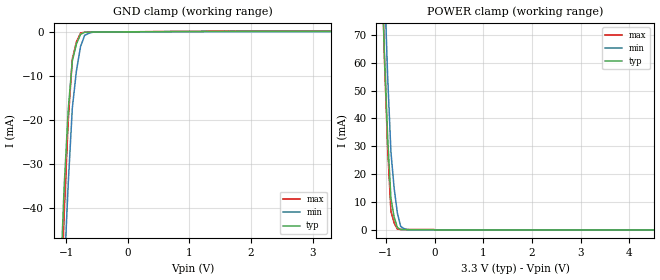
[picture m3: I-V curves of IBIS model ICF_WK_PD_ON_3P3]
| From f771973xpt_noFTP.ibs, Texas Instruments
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|   Model Cell ICF_WK_PD_ON_3P3
|ICF_WK_PD_ON_3P3
[Model]   ICF_WK_PD_ON_3P3
Model_type   Input
Polarity   Non-Inverting
Vinl =  0.8
Vinh =  2
C_comp   0.705929p   0.524756p   0.819798p
[Model Spec]
Vinl   0.8   0.8   0.8
Vinh   2   2   2
[Temperature Range]   25   155   -40
[Voltage Range]   3.3   2.97   3.63
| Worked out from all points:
|   GND clamp passes 1 mA (typ) near -0.78 V on its own axis
|   POWER clamp passes 1 mA (typ) near -0.77 V on its own axis
| Nom Voltages:
|   BIASFET=3.3, VDD=1.2, VDDS=3.3, VSS=0
| Min Voltages:
|   BIASFET=2.97, VDD=1.08, VDDS=2.97, VSS=0
| Max Voltages:
|   BIASFET=3.63, VDD=1.32, VDDS=3.63, VSS=0
[POWER_clamp]
|   voltage   I(typ)   I(min)   I(max)
-3.3V     1.823A     2.351A     1.96A
-1.1V     100.7mA    129.7mA    104mA
-1.033V   62.87mA    88.79mA    61.41mA
-966.7mV  33.08mA    54.88mA    28.95mA
-900mV    11.36mA    27.99mA    6.655mA
-833.3mV  4.591mA    14.88mA    2.454mA
-766.7mV  850.2uA    5.974mA    296.5uA
-700mV    142.4uA    1.28mA     181.4uA
-566.7mV  108.3uA    127.8uA    179.2uA
-500mV    107.6uA    60.24uA    179.1uA
6.6V      0A         0A         0A
[GND_clamp]
|   voltage   I(typ)   I(min)   I(max)
-3.3V     -1.38A     -1.323A    -2.074A
-1.1V     -59.6mA    -79.12mA   -70.72mA
-1.033V   -35.49mA   -55.25mA   -41.83mA
-966.7mV  -17.83mA   -34.66mA   -20.31mA
-900mV    -6.601mA   -17.33mA   -6.147mA
-833.3mV  -2.744mA   -8.865mA   -2.295mA
-766.7mV  -576.6uA   -3.351mA   -278.5uA
-700mV    -97.45uA   -787.6uA   -98.32uA
-566.7mV  -53.29uA   -89.33uA   -76.73uA
3.3V      107.2uA    51.38uA    177.9uA
